| Teraspeed Modeling Services.
| http://www.teraspeed.com
[IBIS Ver]   3.2
[Comment Char] |_char
[File Name]   lpc3152_s4.ibs
[File Rev]   3.0
[Source]  Measured and created by Teraspeed Consulting Group LLC
[Date]   05-04-2010
[Notes]   Quality Check of this IBIS model: Model Passes IBIS Check
   Model parses into ICX IS. Simulation done with Hyperlynx.
   1. MIN TYP MAX information is based on Temperature and Voltage
   characteristics only.
   2. Package data measured using Tektronix IConnect Software.
[Disclaimer]
| Use: Teraspeed Consulting Group LLC ("Teraspeed") has
| licensed IBIS models to specific integrated circuit
| suppliers ("IC Vendors") for use and distribustion as
| follows: Each IC Vendor may use IBIS Models, and distribute
| them to IC Vendor's custumers to use solely for developing
| printed circute board designs. Users of this model may
| modify the IBIS model to suit its specific applications but
| rights to derivative works and such modifications shall belong
| to Teraspeed. No other distribution of these materials is
| permitted.
| DISCLAIMER OF WARRANTY: UNLESS OTHERWISE AGREED TO IN WRITING
| TERASPEED DISCLAIMS AND USER WAIVES ALL WARRANTIES, EXPRESS
| OR IMPLIED, INCLUDING WARRANTIES OF MERCHANTABILITY AND
| FITNESS FOR A PARTICULAR PURPOSE. IN NO EVENT SHALL
| TERASPEED BE LIABLE FOR ANY DIRECT OR INDIRECT DAMAGES,
| WHETHER IN CONTRACT OR TORT, INCLUDING, WITHOUT LIMITATION,
| LOST PROFITS, BUSINESS INTERRUPTION, OR LOST INFORMATION
| ARISING OUT OF THE USE OF OR THE INABILITY TO USE THE MODEL,
| EVEN IF TERASPEED HAS BEEN ADVISED OF THE POSSIBILITY OF SUCH
| DAMAGES.
[Copyright]
| This file is the legal property of Teraspeed Copyright(c) 2010.
| All other rights are reserved.
[Component] LPC3152_S4
[Manufacturer] NXP Semiconductors
[Package]
| variable   typ   min   max
R_pkg  1.000E-02  1.000E-02  1.000E-02
L_pkg  1.600E-09  1.080E-09  3.038E-09
C_pkg  5.473E-13  4.190E-13  9.864E-13
[Pin] signal_name  model_name  R_pin  L_pin C_pin
A1   NC   NC   1.000E-02  1.080E-09  4.190E-13
A2   EBI_A_1_CLE   dio4_s4_out   1.000E-02  2.855E-09  9.268E-13
A3   EBI_D_9   dio4_s4_io   1.000E-02  2.685E-09  8.719E-13
A4   VDDE_IOC   POWER   1.000E-02  1.080E-09  4.190E-13
A5   VSSE_IOC   GND   1.000E-02  1.080E-09  4.190E-13
A6   VDDI   POWER   1.000E-02  1.080E-09  4.190E-13
A7   VSSI   GND   1.000E-02  1.080E-09  4.190E-13
A8   SPI_MISO   dio4_io_3.3v  1.000E-02  2.165E-09  7.029E-13
A9   I2C_SCL0   input   1.000E-02  2.148E-09  6.975E-13
A10  FFAST_IN   osc_in   1.000E-02  2.165E-09  7.029E-13
A11  NC   NC   1.000E-02  1.080E-09  4.190E-13
A12  NC   NC   1.000E-02  1.080E-09  4.190E-13
A13  ADC10B_GNDA   GND   1.000E-02  1.080E-09  4.190E-13
A14  VSSE_IOC   GND   1.000E-02  1.080E-09  4.190E-13
A15  VDDE_IOC   POWER   1.000E-02  1.080E-09  4.190E-13
A16  HP_VDDA33   POWER   1.000E-02  1.080E-09  4.190E-13
A17  NC   NC   1.000E-02  1.080E-09  4.190E-13
B1   NC   NC   1.000E-02  1.080E-09  4.190E-13
B2   NC   NC   1.000E-02  1.080E-09  4.190E-13
B3   NC   NC   1.000E-02  1.080E-09  4.190E-13
B4   NC   NC   1.000E-02  1.080E-09  4.190E-13
B5   mNAND_RYBN0   input   1.000E-02  2.165E-09  7.029E-13
B6   mGPIO9   dio4_io_3.3v  1.000E-02  2.045E-09  6.640E-13
B7   mGPIO6   dio4_io_3.3v  1.000E-02  1.955E-09  6.347E-13
B8   SPI_MOSI   dio4_io_3.3v  1.000E-02  1.899E-09  6.165E-13
B9   NC   NC   1.000E-02  1.080E-09  4.190E-13
B10  FFAST_OUT   osc_out   1.000E-02  1.899E-09  6.165E-13
B11  VDDA12   POWER   1.000E-02  1.080E-09  4.190E-13
B12  ADC10B_GPA0   term   1.000E-02  2.045E-09  6.640E-13
B13  ADC10B_VDDA33   POWER   1.000E-02  1.080E-09  4.190E-13
B14  NC   NC   1.000E-02  1.080E-09  4.190E-13
B15  HP_FCR   term   1.000E-02  2.476E-09  8.038E-13
B16  HP_GNDA   GND   1.000E-02  1.080E-09  4.190E-13
B17  HP_OUTL   term   1.000E-02  2.855E-09  9.268E-13
C1   NC   NC   1.000E-02  1.080E-09  4.190E-13
C2   EBI_D_10   dio4_s4_io   1.000E-02  2.476E-09  8.038E-13
C3   NC   NC   1.000E-02  1.080E-09  4.190E-13
C4   EBI_A_0_ALE   dio4_s4_out   1.000E-02  2.097E-09  6.809E-13
C5   mNAND_RYBN1   input   1.000E-02  1.936E-09  6.287E-13
C6   mGPIO10   dio4_io_3.3v  1.000E-02  1.801E-09  5.849E-13
C7   mGPIO7   dio4_io_3.3v  1.000E-02  1.698E-09  5.514E-13
C8   SPI_SCK   dio4_io_3.3v  1.000E-02  1.633E-09  5.303E-13
C9   VPP   POWER   1.000E-02  1.080E-09  4.190E-13
C10  I2C_SDA0   input   1.000E-02  1.633E-09  5.303E-13
C11  VSSA12   GND   1.000E-02  1.080E-09  4.190E-13
C12  ADC10B_GPA2   term   1.000E-02  1.801E-09  5.849E-13
C13  ADC10B_GPA1   term   1.000E-02  1.936E-09  6.287E-13
C14  DAC_VDDA33   POWER   1.000E-02  1.080E-09  4.190E-13
C15  HP_OUTR   term   1.000E-02  2.279E-09  7.398E-13
C16  HP_FCL   term   1.000E-02  2.476E-09  8.038E-13
C17  PSU_PLAY   term   1.000E-02  2.685E-09  8.719E-13
D1   VDDE_IOA   POWER   1.000E-02  1.080E-09  4.190E-13
D2   EBI_D_11   dio4_s4_io   1.000E-02  2.310E-09  7.500E-13
D3   EBI_D_8   dio4_s4_io   1.000E-02  2.097E-09  6.809E-13
D4   mNAND_RYBN3   input   1.000E-02  1.899E-09  6.165E-13
D5   mNAND_RYBN2   input   1.000E-02  1.719E-09  5.583E-13
D6   mGPIO8   dio4_io_3.3v  1.000E-02  1.566E-09  5.084E-13
D7   mGPIO5   dio4_io_3.3v  1.000E-02  1.446E-09  4.695E-13
D8   SPI_CS_OUT0   dio4_out_3.3v 1.000E-02  1.369E-09  4.446E-13
D9   SPI_CS_IN   input   1.000E-02  1.343E-09  4.359E-13
D10  PWM_DATA_GPIO   dio1_io   1.000E-02  1.369E-09  4.446E-13
D11  GPIO4   input   1.000E-02  1.446E-09  4.695E-13
D12  GPIO3   dio1_io   1.000E-02  1.566E-09  5.084E-13
D13  NC   NC   1.000E-02  1.080E-09  4.190E-13
D14  HP_OUTC   term   1.000E-02  1.899E-09  6.165E-13
D15  PSU_STOP   term   1.000E-02  2.097E-09  6.809E-13
D16  PSU_VSSA   GND   1.000E-02  1.080E-09  4.190E-13
D17  PSU_VSSA_CLEAN   GND   1.000E-02  1.080E-09  4.190E-13
E1   VSSE_IOA   GND   1.000E-02  1.080E-09  4.190E-13
E2   EBI_D_12   dio4_s4_io   1.000E-02  2.165E-09  7.029E-13
E3   EBI_D_7   dio4_s4_io   1.000E-02  1.936E-09  6.287E-13
E4   EBI_D_6   dio4_s4_io   1.000E-02  1.719E-09  5.583E-13
E14  HP_VREF   POWER   1.000E-02  1.080E-09  4.190E-13
E15  RSTIN_N   input   1.000E-02  1.936E-09  6.287E-13
E16  PSU_VBAT   POWER   1.000E-02  1.080E-09  4.190E-13
E17  PSU_VOUT3   term   1.000E-02  2.402E-09  7.798E-13
F1   NC   NC   1.000E-02  1.080E-09  4.190E-13
F2   EBI_D_13   dio4_s4_io   1.000E-02  2.045E-09  6.640E-13
F3   EBI_D_5   dio4_s4_io   1.000E-02  1.801E-09  5.849E-13
F4   EBI_D_4   dio4_s4_io   1.000E-02  1.566E-09  5.084E-13
F14  TDO   dio2_tri   1.000E-02  1.566E-09  5.084E-13
F15  DAC_VREFN   POWER   1.000E-02  1.080E-09  4.190E-13
F16  DAC_VREFP   POWER   1.000E-02  1.080E-09  4.190E-13
F17  PSU_VBAT2   POWER   1.000E-02  1.080E-09  4.190E-13
G1   NC   NC   1.000E-02  1.080E-09  4.190E-13
G2   EBI_D_14   dio4_s4_io   1.000E-02  1.955E-09  6.347E-13
G3   NC   NC   1.000E-02  1.080E-09  4.190E-13
G4   EBI_D_3   dio4_s4_io   1.000E-02  1.446E-09  4.695E-13
G14  PSU_VOUT2   term   1.000E-02  1.446E-09  4.695E-13
G15  VDDE_IOD   POWER   1.000E-02  1.080E-09  4.190E-13
G16  PSU_VIN1   term   1.000E-02  1.955E-09  6.347E-13
G17  PSU_LX2   term   1.000E-02  2.214E-09  7.190E-13
H1   VSSI   GND   1.000E-02  1.080E-09  4.190E-13
H2   EBI_D_15   dio4_s4_io   1.000E-02  1.899E-09  6.165E-13
H3   EBI_D_1   dio4_s4_io   1.000E-02  1.633E-09  5.303E-13
H4   EBI_D_2   dio4_s4_io   1.000E-02  1.369E-09  4.446E-13
H14  PSU_VOUT1   term   1.000E-02  1.369E-09  4.446E-13
H15  PSU_LX1   term   1.000E-02  1.633E-09  5.303E-13
H16  PSU_VSS1   GND   1.000E-02  1.080E-09  4.190E-13
H17  PSU_VBAT1   POWER   1.000E-02  1.080E-09  4.190E-13
J1   VDDI   POWER   1.000E-02  1.080E-09  4.190E-13
J2   EBI_NCAS_BLOUT_0 dio4_s4_out   1.000E-02  1.880E-09  6.103E-13
J3   EBI_D_0   dio4_s4_io   1.000E-02  1.611E-09  5.231E-13
J4   EBI_NRAS_BLOUT_1 dio4_s4_out   1.000E-02  1.343E-09  4.359E-13
J14  CHARGE_VBUS   POWER   1.000E-02  1.080E-09  4.190E-13
J15  CHARGE_VSS   GND   1.000E-02  1.080E-09  4.190E-13
J16  PSU_VBUS   POWER   1.000E-02  1.080E-09  4.190E-13
J17  CHARGE_VNTC   term   1.000E-02  2.148E-09  6.975E-13
K1   VSSE_IOB   GND   1.000E-02  1.080E-09  4.190E-13
K2   NC   NC   1.000E-02  1.080E-09  4.190E-13
K3   EBI_DQM_0_NOE   dio4_s4_out   1.000E-02  1.633E-09  5.303E-13
K4   EBI_NWE   dio4_s4_out   1.000E-02  1.369E-09  4.446E-13
K14  RTC_BACKUP   POWER   1.000E-02  1.080E-09  4.190E-13
K15  CHARGE_CC_REF   POWER   1.000E-02  1.080E-09  4.190E-13
K16  CHARGE_VBAT   POWER   1.000E-02  1.080E-09  4.190E-13
K17  CHARGE_BAT_SENSE term   1.000E-02  2.165E-09  7.029E-13
L1   VDDE_IOB   POWER   1.000E-02  1.080E-09  4.190E-13
L2   NAND_NCS_0   dio4_s4_out   1.000E-02  1.955E-09  6.347E-13
L3   NAND_NCS_1   dio4_s4_out   1.000E-02  1.698E-09  5.514E-13
L4   NAND_NCS_2   dio4_s4_out   1.000E-02  1.446E-09  4.695E-13
L14  VSSE_IOD   GND   1.000E-02  1.080E-09  4.190E-13
L15  RTC_VDD36   POWER   1.000E-02  1.080E-09  4.190E-13
L16  FSLOW_OUT   osc_out   1.000E-02  1.955E-09  6.347E-13
L17  FSLOW_IN   osc_in   1.000E-02  2.214E-09  7.190E-13
M1   VDDE_IOA   POWER   1.000E-02  1.080E-09  4.190E-13
M2   NAND_NCS_3   dio4_s4_out   1.000E-02  2.045E-09  6.640E-13
M3   NC   NC   1.000E-02  1.080E-09  4.190E-13
M4   CLOCK_OUT   dio4_s4_out   1.000E-02  1.566E-09  5.084E-13
M14  VDDI_AD   POWER   1.000E-02  1.080E-09  4.190E-13
M15  VSSI_AD   GND   1.000E-02  1.080E-09  4.190E-13
M16  RTC_INT   osc_out   1.000E-02  2.045E-09  6.640E-13
M17  RTC_VSS   GND   1.000E-02  1.080E-09  4.190E-13
N1   VSSE_IOA   GND   1.000E-02  1.080E-09  4.190E-13
N2   USB_VDDA12_PLL   POWER   1.000E-02  1.080E-09  4.190E-13
N3   USB_VBUS   POWER   1.000E-02  1.080E-09  4.190E-13
N4   USB_RREF   term   1.000E-02  1.719E-09  5.583E-13
N14  ADC_VDDA33   POWER   1.000E-02  1.080E-09  4.190E-13
N15  ADC_VDDA18   POWER   1.000E-02  1.080E-09  4.190E-13
N16  ADC_GNDA   GND   1.000E-02  1.080E-09  4.190E-13
N17  UOS_VSS   GND   1.000E-02  1.080E-09  4.190E-13
P1   NC   NC   1.000E-02  1.080E-09  4.190E-13
P2   USB_VSSA_REF   GND   1.000E-02  1.080E-09  4.190E-13
P3   USB_ID   term   1.000E-02  2.097E-09  6.809E-13
P4   mLCD_DB_10   dio4_s8_io   1.000E-02  1.899E-09  6.165E-13
P5   mLCD_DB_9   dio4_s8_io   1.000E-02  1.719E-09  5.583E-13
P6   mLCD_DB_5   dio4_s8_io   1.000E-02  1.566E-09  5.084E-13
P7   mLCD_E_RD   dio4_s8_out   1.000E-02  1.446E-09  4.695E-13
P8   mLCD_DB_1   dio4_s8_io   1.000E-02  1.369E-09  4.446E-13
P9   I2SRX_DATA0_GPIO dio1_io   1.000E-02  1.343E-09  4.359E-13
P10  UART_TXD_GPIO   dio1_io   1.000E-02  1.369E-09  4.446E-13
P11  mUART_CTS_N_GPIO dio1_io   1.000E-02  1.446E-09  4.695E-13
P12  GPIO2   dio1_io   1.000E-02  1.566E-09  5.084E-13
P13  ADC_TINL   term   1.000E-02  1.719E-09  5.583E-13
P14  ADC_TINR   term   1.000E-02  1.899E-09  6.165E-13
P15  UOS_VBUS   POWER   1.000E-02  1.080E-09  4.190E-13
P16  UOS_VBAT   POWER   1.000E-02  1.080E-09  4.190E-13
P17  UOS_CX2   term   1.000E-02  2.533E-09  8.225E-13
R1   USB_DM   term   1.000E-02  2.685E-09  8.719E-13
R2   USB_VSSA_TERM   GND   1.000E-02  1.080E-09  4.190E-13
R3   USB_VDDA33   POWER   1.000E-02  1.080E-09  4.190E-13
R4   mLCD_DB_15   dio4_s8_io   1.000E-02  2.097E-09  6.809E-13
R5   mLCD_DB_6   dio4_s8_io   1.000E-02  1.936E-09  6.287E-13
R6   mLCD_DB_3   dio4_s8_io   1.000E-02  1.801E-09  5.849E-13
R7   mLCD_RS   dio4_s8_out   1.000E-02  1.698E-09  5.514E-13
R8   mLCD_CSB   dio4_s8_out   1.000E-02  1.633E-09  5.303E-13
R9   I2SRX_WS0_GPIO   dio1_io   1.000E-02  1.611E-09  5.231E-13
R10  UART_RXD_GPIO   dio1_io   1.000E-02  1.633E-09  5.303E-13
R11  mUART_RTS_N_GPIO dio1_io   1.000E-02  1.698E-09  5.514E-13
R12  mI2STX_WS0_GPIO  dio1_io   1.000E-02  1.801E-09  5.849E-13
R13  GPIO0   dio1_io   1.000E-02  1.936E-09  6.287E-13
R14  ADC_VINR   term   1.000E-02  2.097E-09  6.809E-13
R15  ADC_MIC   term   1.000E-02  2.279E-09  7.398E-13
R16  ADC_VREFN   POWER   1.000E-02  1.080E-09  4.190E-13
R17  UOS_CX1   term   1.000E-02  2.685E-09  8.719E-13
T1   USB_DP   term   1.000E-02  2.855E-09  9.268E-13
T2   USB_GNDA   GND   1.000E-02  1.080E-09  4.190E-13
T3   USB_VDDA33_DRV   POWER   1.000E-02  1.080E-09  4.190E-13
T4   mLCD_DB_12   dio4_s8_io   1.000E-02  2.310E-09  7.500E-13
T5   mLCD_DB_7   dio4_s8_io   1.000E-02  2.165E-09  7.029E-13
T6   mLCD_DB_2   dio4_s8_io   1.000E-02  2.045E-09  6.640E-13
T7   mLCD_DB_0   dio4_s8_io   1.000E-02  1.955E-09  6.347E-13
T8   mLCD_RW_WR   dio4_s8_out   1.000E-02  1.899E-09  6.165E-13
T9   I2SRX_BCK0_GPIO  dio1_io   1.000E-02  1.880E-09  6.103E-13
T10  TDI_GPIO   dio1_io   1.000E-02  1.899E-09  6.165E-13
T11  mI2STX_CLK0_GPIO dio1_io   1.000E-02  1.955E-09  6.347E-13
T12  mI2STX_BCK0_GPIO dio1_io   1.000E-02  2.045E-09  6.640E-13
T13  mI2STX_DAT0_GPIO dio1_io   1.000E-02  2.165E-09  7.029E-13
T14  GPIO1   dio1_io   1.000E-02  2.310E-09  7.500E-13
T15  ADC_VINL   term   1.000E-02  2.476E-09  8.038E-13
T16  ADC_VREF   POWER   1.000E-02  1.080E-09  4.190E-13
T17  ADC_VREFP   POWER   1.000E-02  1.080E-09  4.190E-13
U1   NC   NC   1.000E-02  1.080E-09  4.190E-13
U2   mLCD_DB_14   dio4_s8_io   1.000E-02  2.855E-09  9.268E-13
U3   mLCD_DB_13   dio4_s8_io   1.000E-02  2.685E-09  8.719E-13
U4   mLCD_DB_11   dio4_s8_io   1.000E-02  2.533E-09  8.225E-13
U5   mLCD_DB_8   dio4_s8_io   1.000E-02  2.402E-09  7.798E-13
U6   mLCD_DB_4   dio4_s8_io   1.000E-02  2.294E-09  7.449E-13
U7   VDDE_IOB   POWER   1.000E-02  1.080E-09  4.190E-13
U8   VSSE_IOB   GND   1.000E-02  1.080E-09  4.190E-13
U9   TMS_GPIO   dio1_io   1.000E-02  2.148E-09  6.975E-13
U10  JTAGSEL_GPIO   dio1_io   1.000E-02  2.165E-09  7.029E-13
U11  TRST_N_GPIO   dio1_io   1.000E-02  2.214E-09  7.190E-13
U12  TCK_GPIO   dio1_io   1.000E-02  2.294E-09  7.449E-13
U13  VDDI   POWER   1.000E-02  1.080E-09  4.190E-13
U14  VSSI   GND   1.000E-02  1.080E-09  4.190E-13
U15  VDDE_IOC   POWER   1.000E-02  1.080E-09  4.190E-13
U16  VSSE_IOC   GND   1.000E-02  1.080E-09  4.190E-13
U17  RTC_CLK32   osc_out   1.000E-02  3.038E-09  9.864E-13
[Model Selector]  dio4_s4_io
dio4_io_1.8v   dio4_io, sup4=1.8v
dio4_io_3.3v   dio4_io, sup4=3.3v
[Model Selector]  dio4_s4_out
dio4_out_1.8v  dio4_out, sup4=1.8v
dio4_out_3.3v  dio4_out, sup4=3.3v
[Model Selector]  dio4_s8_io
dio4_io_1.8v   dio4_io, sup8=1.8v
dio4_io_3.3v   dio4_io, sup8=3.3v
[Model Selector]  dio4_s8_out
dio4_out_1.8v  dio4_out, sup8=1.8v
dio4_out_3.3v  dio4_out, sup8=3.3v
[Model] term
Model_type Terminator
C_comp  0pF 0pF 0pF
| variable typ   min   max
[Voltage Range]   3.30000V  3.00000V  3.60000V
[POWER Clamp Reference]  3.30000V  3.00000V  3.60000V
[GND Clamp Reference]   0.00000V  0.00000V  0.00000V
[Temperature Range]   25   85   -40
| Models and submodels in the file (10): input (Input), dio1_io (I/O), dio2_tri (3-state), dio4_io_1.8v (I/O), dio4_io_3.3v (I/O), dio4_out_1.8v (Output), dio4_out_3.3v (Output), osc_in (Input), osc_out (Output), term (Terminator)
